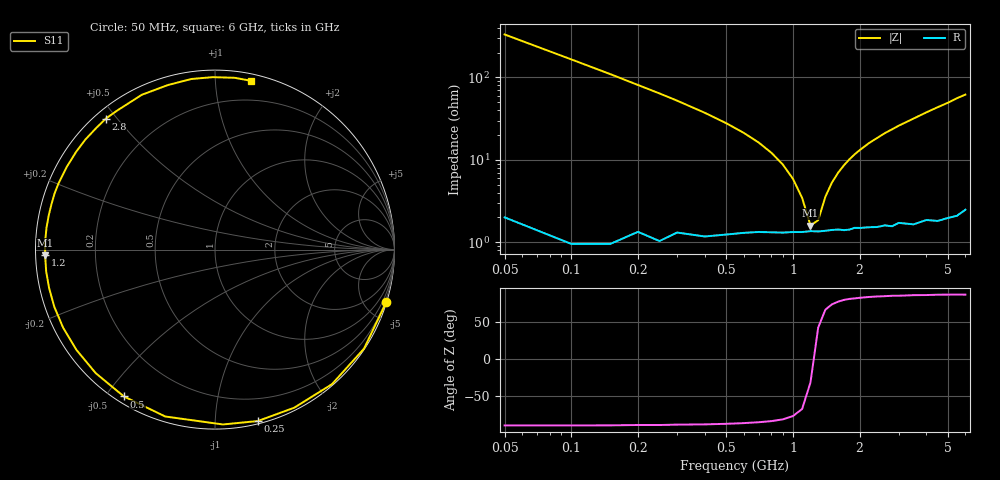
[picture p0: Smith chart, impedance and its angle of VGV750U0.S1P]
! Infineon Technologies  Discrete & RF Semiconductors
! BB 831
! Si Tuning Diode in SOD323
! VR = 0.75 V
! S-Parameters:  July  1999
# GHz  S  MA  R  50
!  f  S11
! GHz  MAG  ANG
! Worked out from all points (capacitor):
!   34 points, 50 MHz to 6 GHz, reference 50 ohm
!   read as one part to ground: C = 9.55 pF near 50 MHz
!   lowest |Z| = 1.59 ohm at 1.2 GHz (marker M1)
!   series resonance near 1.24 GHz, so ESL is about 1.7 nH
!   S11 on the Smith chart (normalised r, x): 50 MHz: 0.04, -6.65; 250 MHz: 0.02, -1.28; 500 MHz: 0.02, -0.56; 1.2 GHz: 0.03, -0.02; 2.8 GHz: 0.03, +0.47; 6 GHz: 0.05, +1.24
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0.05  0.9982 -17.1
0.1  0.9968 -33.6
0.15  0.9935 -49.0
0.2  0.9853 -63.4
0.25  0.9845 -76.0
0.3  0.9753 -87.4
0.4  0.9703 -106.6
0.5  0.9628 -121.8
0.6  0.9569 -134.0
0.7  0.9529 -144.1
0.8  0.9514 -152.8
0.9  0.9504 -160.3
1  0.9489 -166.9
1.2  0.947 -178.1
1.4  0.9466 172.5
1.6  0.9455 164.4
1.8  0.9467 157.2
2  0.9457 150.8
2.2  0.9463 144.8
2.4  0.9475 139.6
2.8  0.9501 129.8
3  0.9473 125.2
3.5  0.954 115.3
4  0.9536 106.0
4.5  0.9596 97.9
5  0.9608 90.8
5.5  0.9635 83.5
6  0.9617 77.8
